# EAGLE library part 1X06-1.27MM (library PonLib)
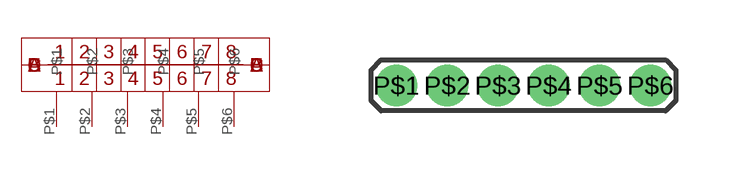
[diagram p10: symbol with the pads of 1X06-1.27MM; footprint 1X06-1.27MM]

Designator prefix -

## 1X06-1.27MM  [1X06-1.27MM]
P$1  P$1
P$2  P$2
P$3  P$3
P$4  P$4
P$5  P$5
P$6  P$6

## Footprint 1X06-1.27MM (pad centres in mm)
drill 0.533 pad 0.889: P$1 -3.175,0; P$2 -1.905,0; P$3 -0.635,0; P$4 0.635,0; P$5 1.905,0; P$6 3.175,0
